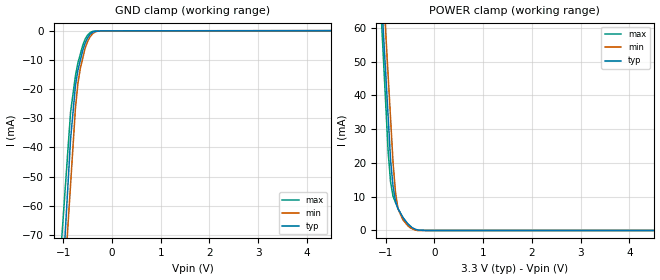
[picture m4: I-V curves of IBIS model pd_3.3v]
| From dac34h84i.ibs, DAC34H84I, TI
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[Model] pd_3.3v
Model_type Input
Vinl = 990.000mV
Vinh = 2.31000V
C_comp 1.63000pF 1.63000pF 1.63000pF
| variable typ   min   max
[Voltage Range] 3.30000V 3.00000V 3.60000V
[POWER Clamp Reference] 3.30000V 3.00000V 3.60000V
[GND Clamp Reference] 0.00000V 0.00000V 0.00000V
[Temperature Range] 25   125   -40
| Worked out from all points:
|   GND clamp passes 1 mA (typ) near -0.43 V on its own axis
|   POWER clamp passes 1 mA (typ) near -0.47 V on its own axis
[GND Clamp]
-3.3V     -756.2mA   -694.8mA   -612.9mA
-850mV    -37.07mA   -52.65mA   -27.84mA
-750mV    -18.8mA    -26.44mA   -15.45mA
-700mV    -13.6mA    -18.06mA   -11.08mA
-650mV    -10.16mA   -12.9mA    -8.012mA
-600mV    -6.706mA   -9.374mA   -4.946mA
-550mV    -4.203mA   -5.845mA   -2.837mA
-500mV    -2.418mA   -3.65mA    -1.45mA
-400mV    -534.9uA   -1.05mA    -226.8uA
-300mV    -145.6uA   -173.5uA   -53.62uA
-150mV    -16.29uA   -18.92uA   -17.23uA
6.6V      55.69uA    64.66uA    46.36uA
[POWER Clamp]
-3.3V     635mA      646.2mA    690.2mA
-1.15V    84.53mA    96.64mA    79.81mA
-1.05V    58.92mA    71.08mA    51.42mA
-950mV    33.32mA    45.52mA    23.03mA
-900mV    20.52mA    32.74mA    14.17mA
-850mV    13.01mA    19.96mA    10.09mA
-800mV    8.674mA    11.25mA    8.269mA
-750mV    6.513mA    6.481mA    6.452mA
-650mV    3.883mA    3.184mA    3.807mA
-500mV    1.366mA    811.6uA    1.24mA
-400mV    438.6uA    132.6uA    231.9uA
6.6V      0A         0A         0A
